// TwinCAT 3 PLC project PLCProject
// ProgramVersion: 3.1.4024.0
// libraries:
//   Tc2_Standard, * (Beckhoff Automation GmbH)
//   Tc2_System, * (Beckhoff Automation GmbH)
//   Tc2_Utilities, * (Beckhoff Automation GmbH)
//   Tc3_EventLogger, * (Beckhoff Automation GmbH)
//   Tc3_Module, * (Beckhoff Automation GmbH)
// project tree:
//   DUTs/ ST_event.TcDUT, ST_recept.TcDUT
//   / PlcTask.TcTTO
//   POUs/ AlarmsAndEvents.TcPOU, AlarmsAndEventsCX7000.TcPOU, EventController.TcPOU, MAIN.TcPOU
// real-time tasks:
//   TASK PlcTask: cycle T#10ms, priority 20, ADS port 350
// I/O:
//   DEVICE Device 3 (CX7000) (disabled), AmsNetId 172.16.3.128.4.1
//     Term 1 (CX7028) [CX7028-0000-0118]
//       modules: Module 1 (DIO_2x), Module 3 (DIO_2x), Module 5 (DI_2x), Module 7 (DI_2x)
//   DEVICE Device 1 (EtherCAT) (disabled), AmsNetId 172.16.3.128.2.1
//     Term 1 (EK1200) [EK1200-7000 EtherCAT Power supply (1,5A E-Bus)]
//       Term 2 (EL1859) [EL1859 8Ch. Dig. Input 24V, 3ms, 8Ch. Dig. Output 24V, 0.5A]
//       Term 3 (EL1859) [EL1859 8Ch. Dig. Input 24V, 3ms, 8Ch. Dig. Output 24V, 0.5A]
//       Term 4 (EL9011) [EL9011 End Terminal]

CONFIGURATION PLCProject
    RESOURCE PLC ON TwinCAT3
        TASK PlcTask(INTERVAL := T#10ms, PRIORITY := 20);
        PROGRAM MAIN WITH PlcTask : MAIN;
    END_RESOURCE
END_CONFIGURATION

// ---- DUTs/ST_event.TcDUT
TYPE ST_event :
STRUCT
	severity : INT := 0; // 0 - info, 1 - warning, 2 - error, 3 - critical
	state : INT := 0; // 0 - inactive, 1 - raised, 2 - confirmed, 3 - active (non-confirmable)
	needs_confirmation : BOOL := FALSE; // FALSE: INACTIVE -> ACTIVE; we go to INACTIVE after received clear action; TRUE: when in state RAISED, we go to CONFIRMED after confirm action, and then to INACTIVE after clear
	timestamp_raised : DATE_AND_TIME; // When event was raised
	timestamp_confirmed : DATE_AND_TIME; // When event was confirmed
	display_text : STRING(255) := '';
	cause_text : STRING(255) := '';
	remedy_text : STRING(255) := '';	
END_STRUCT
END_TYPE

// ---- DUTs/ST_recept.TcDUT
TYPE ST_recept :
STRUCT
	modra : INT := 50;
	rdeca : INT := 20;
	zelena: INT := 0;
	voda: INT := 10;
END_STRUCT
END_TYPE

// ---- POUs/MAIN.TcPOU
PROGRAM MAIN
VAR
	{attribute 'OPC.UA.DA' := '1'}
	{attribute'OPC.UA.DA.Access' := '1'}
	// Access: 0 => no access, 1 => readonly, 2 => writeonly, 3 (default) => rw
	preklopnik: BOOL;
	{attribute 'OPC.UA.DA' := '1'}
	{attribute'OPC.UA.DA.Access' := '3'} 
	{attribute 'OPC.UA.DA.Description' :='ID izdelka'}
	izdelekID: INT;
	{attribute 'OPC.UA.DA' := '1'}
	recept: ST_recept;
END_VAR

AlarmsAndEvents();
AlarmsAndEventsCX7000();

END_PROGRAM

// ---- POUs/AlarmsAndEvents.TcPOU
PROGRAM AlarmsAndEvents
VAR
	isInitialized      : BOOL := FALSE;
	sendInfo           : BOOL := FALSE;
	sendWarning        : BOOL := FALSE;
	raiseAlarmError    : BOOL := FALSE;
	raiseAlarmWarning  : BOOL := FALSE;
	confirmAlarmError  : BOOL;
	clearAlarms        : BOOL;
	fbMessageInfo      : FB_TcMessage;
	fbMessageWarning   : FB_TcMessage;	
	fbAlarmWarning     : FB_TcAlarm;		
	fbAlarmError       : FB_TcAlarm;	
END_VAR

// This code demonstrates usage of EventLogger system for Alarms and Events.
// However, CX7000 PLC is not capable of using EventLogger. Thus we need workarounds. See PRG AlarmsAndEventsCX7000.

IF NOT isInitialized THEN
	isInitialized := TRUE;
	fbMessageInfo.CreateEx(TC_EVENTS.MyEventClass.MyEventInfo, 0);
	fbMessageWarning.CreateEx(TC_EVENTS.MyEventClass.MyEventWarning, 0);
	fbAlarmWarning.CreateEx(TC_EVENTS.MyEventClass.MyEventWarning, 0, 0);
	fbAlarmError.CreateEx(TC_EVENTS.MyEventClass.MyEventError, 1, 0);
END_IF

IF sendInfo THEN
	sendInfo := FALSE;
	fbMessageInfo.Send(0); // 0 - set current timestamp automatically
END_IF

IF sendWarning THEN
	sendWarning := FALSE;
	fbMessageWarning.Send(0);
END_IF

IF raiseAlarmWarning THEN
	raiseAlarmWarning := FALSE;
	fbAlarmWarning.Raise(0);
END_IF

IF raiseAlarmError THEN
	raiseAlarmError := FALSE;
	fbAlarmError.Raise(0);
END_IF

IF confirmAlarmError THEN
	confirmAlarmError := FALSE;
	fbAlarmError.Confirm(0);
END_IF

IF clearAlarms THEN
	clearAlarms := FALSE;
	fbAlarmWarning.Clear(0, TRUE);
	fbAlarmError.Clear(0, TRUE);
END_IF

END_PROGRAM

// ---- POUs/AlarmsAndEventsCX7000.TcPOU
PROGRAM AlarmsAndEventsCX7000
VAR
	events: ARRAY[0..7] OF ST_event;
	fbEvent_0: EventController;
	fbEvent_1: EventController;
	fbEvent_2: EventController;
	fbEvent_3: EventController;
	confirmAll: BOOL;
	clearAll: BOOL;
	resetAll: BOOL;
	initEvents : BOOL := FALSE;
	
END_VAR


IF NOT initEvents THEN
	initEvents := TRUE;
	
	// Info message
	events[0].severity := 0;
	events[0].needs_confirmation := FALSE;
	events[0].display_text := 'Nov izdelek na vhodnem traku.';
	events[0].cause_text := 'Prožena je fotocelica na vhodu';
	events[0].remedy_text := '';
	
	// Warning
	events[1].severity := 1;
	events[1].needs_confirmation := FALSE;
	events[1].display_text := 'Končan izdelek čaka na izhodu.';
	events[1].cause_text := 'Prožena je fotocelica na izhodu';
	events[1].remedy_text := 'Odstrani izdelek na izhodu.';
	
	// Error
	events[2].severity := 2;
	events[2].needs_confirmation := TRUE;
	events[2].display_text := 'Potiskač 1 v okvari.';
	events[2].cause_text := 'Aktivni sta obe končni stikali.';
	events[2].remedy_text := 'Preveri končna stikala, javi serviserju.';
	
	// Critical
	events[3].severity := 3;
	events[3].needs_confirmation := TRUE;
	events[3].display_text := 'Prekoračena omejitev iztega.';
	events[3].cause_text := 'Stevec korakov je vecji od dovoljene meje.';
	events[3].remedy_text := 'Prestavi v rocni nacin in referenciraj robota.';
	
END_IF

// Call the event controllers, each for an event
fbEvent_0(eventData := events[0]);
fbEvent_1(eventData := events[1]);
fbEvent_2(eventData := events[2]);
fbEvent_3(eventData := events[3]);

// Confirmation (if required)
fbEvent_2.confirm := confirmAll;
fbEvent_3.confirm := confirmAll;

// Clear
fbEvent_0.clear := clearAll;
fbEvent_1.clear := clearAll;
fbEvent_2.clear := clearAll;
fbEvent_3.clear := clearAll;

// Reset
fbEvent_0.reset := resetAll;
fbEvent_1.reset := resetAll;
fbEvent_2.reset := resetAll;
fbEvent_3.reset := resetAll;

END_PROGRAM

// ---- POUs/EventController.TcPOU
FUNCTION_BLOCK EventController
VAR_IN_OUT
	eventData: ST_event;
END_VAR
VAR_INPUT
	raise: bool;
	confirm: bool;
	clear: bool;
	reset: bool;
END_VAR
VAR
	fbTime: FB_LocalSystemTime := (bEnable := TRUE, dwCycle := 1);
	currTime: TIMESTRUCT;
END_VAR

// FB for state control of an event
// States:
// 0 - INACTIVE
// 1 - RAISED
// 2 - CONFIRMED

// Get current time
fbTime();

IF reset THEN	
	eventData.state := 0;
	eventData.timestamp_raised := DT#1970-1-1-0:0;
	eventData.timestamp_confirmed := DT#1970-1-1-0:0;
	
ELSE
	
	CASE eventData.state OF
		0:  // INACTIVE
			IF raise THEN
				
				currTime := fbTime.systemTime;
				eventData.timestamp_raised := SYSTEMTIME_TO_DT(TIMESTR := currTime);
				IF eventData.needs_confirmation THEN
					eventData.state := 1;
				ELSE
					eventData.state := 3;
				END_IF
			END_IF
		1:  // RAISED (confirmable)
			// If confirmation is needed and we get the confirm signal, we change state to CONFIRMED
			IF confirm THEN
				eventData.state := 2;
				eventData.timestamp_confirmed := SYSTEMTIME_TO_DT(TIMESTR := currTime);
			END_IF
		2:  // CONFIRMED (confirmable)
			// Change state to INACTIVE if clear signal is high and raise is low
			IF clear AND NOT raise THEN
				eventData.state := 0;
			END_IF
		3:  // ACTIVE (non-confirmable)
			// If confirmation is not required, we can clear the event on a high clear input and transit to INACTIVE state
			IF clear AND NOT raise THEN
				eventData.state := 0;
			END_IF
		
		ELSE
			eventData.state := 0;
		
	END_CASE
END_IF

END_FUNCTION_BLOCK
